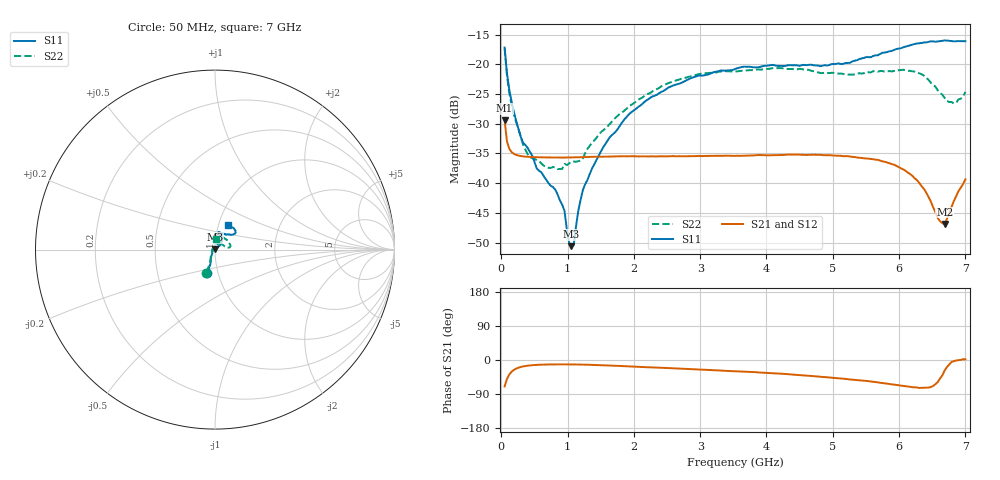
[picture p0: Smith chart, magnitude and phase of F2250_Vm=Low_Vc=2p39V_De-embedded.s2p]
! Integrated Device Technology
! Corporate Headquarters
! 6024 Silver Creek Valley Road
! San Jose, CA 95138  USA
! Phone:  1-408-284-8200
! Toll Free:  1-800-223-1366
! Webpage:  http://www.idt.com/
! Timing and RF Division
! 515 Groton Road, Suite 102
! Westford, MA 01886-6024
! Device:  F2250
! Description: Voltage Variable RF Attenuator
! Frequency:  50.0 -  6000.00 MHz
! Package:  3x3 mm Thin QFN Plastic Package: 16 pin
! Ports:  2 RF, 3 DC
!  Pin  1  = GND
!  Pin  2  = NC
!  Pin  3  = RF1  = Port 1
!  Pin  4  = NC
!  Pin  5  = GND
!  Pin  6  = GND
!  Pin  7  = GND
!  Pin  8  = GND
!  Pin  9  = NC
!  Pin 10  = RF2  = Port 2
!  Pin 11  = NC
!  Pin 12  = GND
!  Pin 13  = GND
!  Pin 14  = VCNTRL
!  Pin 15  = VDD
!  Pin 16  = VMODE
! Vcntrl:  2.390 Volts
! Vmode:  +0.000 Volts
! Vdd:  +3.30  Volts
! Current:  1.175 mA
! Data:  The device was measured on a the F2250 evaluation board which has
!  individual transmission lines to the RF pins.  Data was collected
!  using a calibrated network analyzer.  The evaluation board was
!  de-embedded using a TRL calibration technique.
!  The reference plane is the edge of the package pin.
! Misc:  SN 10
!  Action Tracker AT0258
! Date Measured:  2014-11-26
! Date:  2015-10-15  MJV
! Note:
!  Integrated Device Technology supplies this data as a sample of measured
!  data at the package pin for this product.  Your particular data for this
!  product may vary.
!  Data was taken at 25 degrees C.
!  Integrated Device Technology reserves the right to change this data at anytime.
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# GHz S dB R 50
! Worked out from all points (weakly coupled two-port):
!   201 points, 50 MHz to 7 GHz, reference 50 ohm
!   highest |S21| = -29.41 dB at 50 MHz (marker M1); lowest = -46.9 dB at 6.687 GHz (marker M2)
!   lowest |S11| = -50.6 dB at 1.058 GHz (marker M3), VSWR 1.01, Z = 49.8 + j0.249 ohm
!   |S11| at or under -10 dB: start of sweep to end of sweep
!   |S22| runs from -37.6 to -17.3 dB; largest |S21 - S12| = 5.9e-05
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0.05  -17.18 -108.6  -29.41 -69.8  -29.41 -69.8  -17.28 -111.0
0.08475  -21.45 -107.4  -32.91 -50.3  -32.91 -50.3  -21.76 -110.1
0.15425  -26.23 -116.6  -34.75 -31.1  -34.75 -31.1  -26.83 -122.2
0.29325  -32.21 -127.7  -35.43 -18.5  -35.42 -18.5  -32.14 -137.3
0.3975  -34.07 -141.7  -35.55 -15.0  -35.55 -15.0  -35.11 -160.3
0.91875  -43.59 158.2  -35.67 -11.5  -35.68 -11.5  -37.59 133.1
0.9535  -44.65 169.4  -35.68 -11.5  -35.68 -11.5  -36.74 130.9
1.023  -50.02 144.2  -35.67 -11.6  -35.67 -11.6  -36.67 115.4
1.05775  -50.58 122.4  -35.66 -11.6  -35.66 -11.6  -36.34 110.5
1.0925  -50.39 90.5  -35.65 -11.7  -35.65 -11.7  -36.35 105.7
1.162  -44.60 57.0  -35.63 -11.9  -35.63 -11.9  -36.29 95.0
1.2315  -41.10 44.1  -35.60 -12.1  -35.61 -12.1  -35.82 85.3
1.6485  -32.10 41.9  -35.52 -14.6  -35.51 -14.6  -29.88 64.3
1.96125  -28.05 42.2  -35.46 -17.2  -35.46 -17.2  -26.81 56.7
2.37825  -24.87 47.3  -35.47 -20.3  -35.47 -20.3  -24.00 56.7
3.525  -20.80 72.4  -35.40 -29.5  -35.40 -29.5  -21.20 74.7
4.7065  -20.16 72.3  -35.20 -42.5  -35.20 -42.5  -21.16 72.3
5.85325  -17.81 40.5  -36.63 -63.2  -36.63 -63.3  -21.14 22.9
6.27025  -16.51 40.1  -39.49 -72.5  -39.51 -72.7  -21.36 9.6
6.68725  -15.99 48.8  -46.85 -27.7  -46.83 -27.4  -25.65 28.4
6.861  -16.13 55.1  -42.18 -1.3  -42.13 -1.2  -26.48 58.0
7  -16.13 63.2  -39.34 1.9  -39.31 1.7  -24.63 83.2
